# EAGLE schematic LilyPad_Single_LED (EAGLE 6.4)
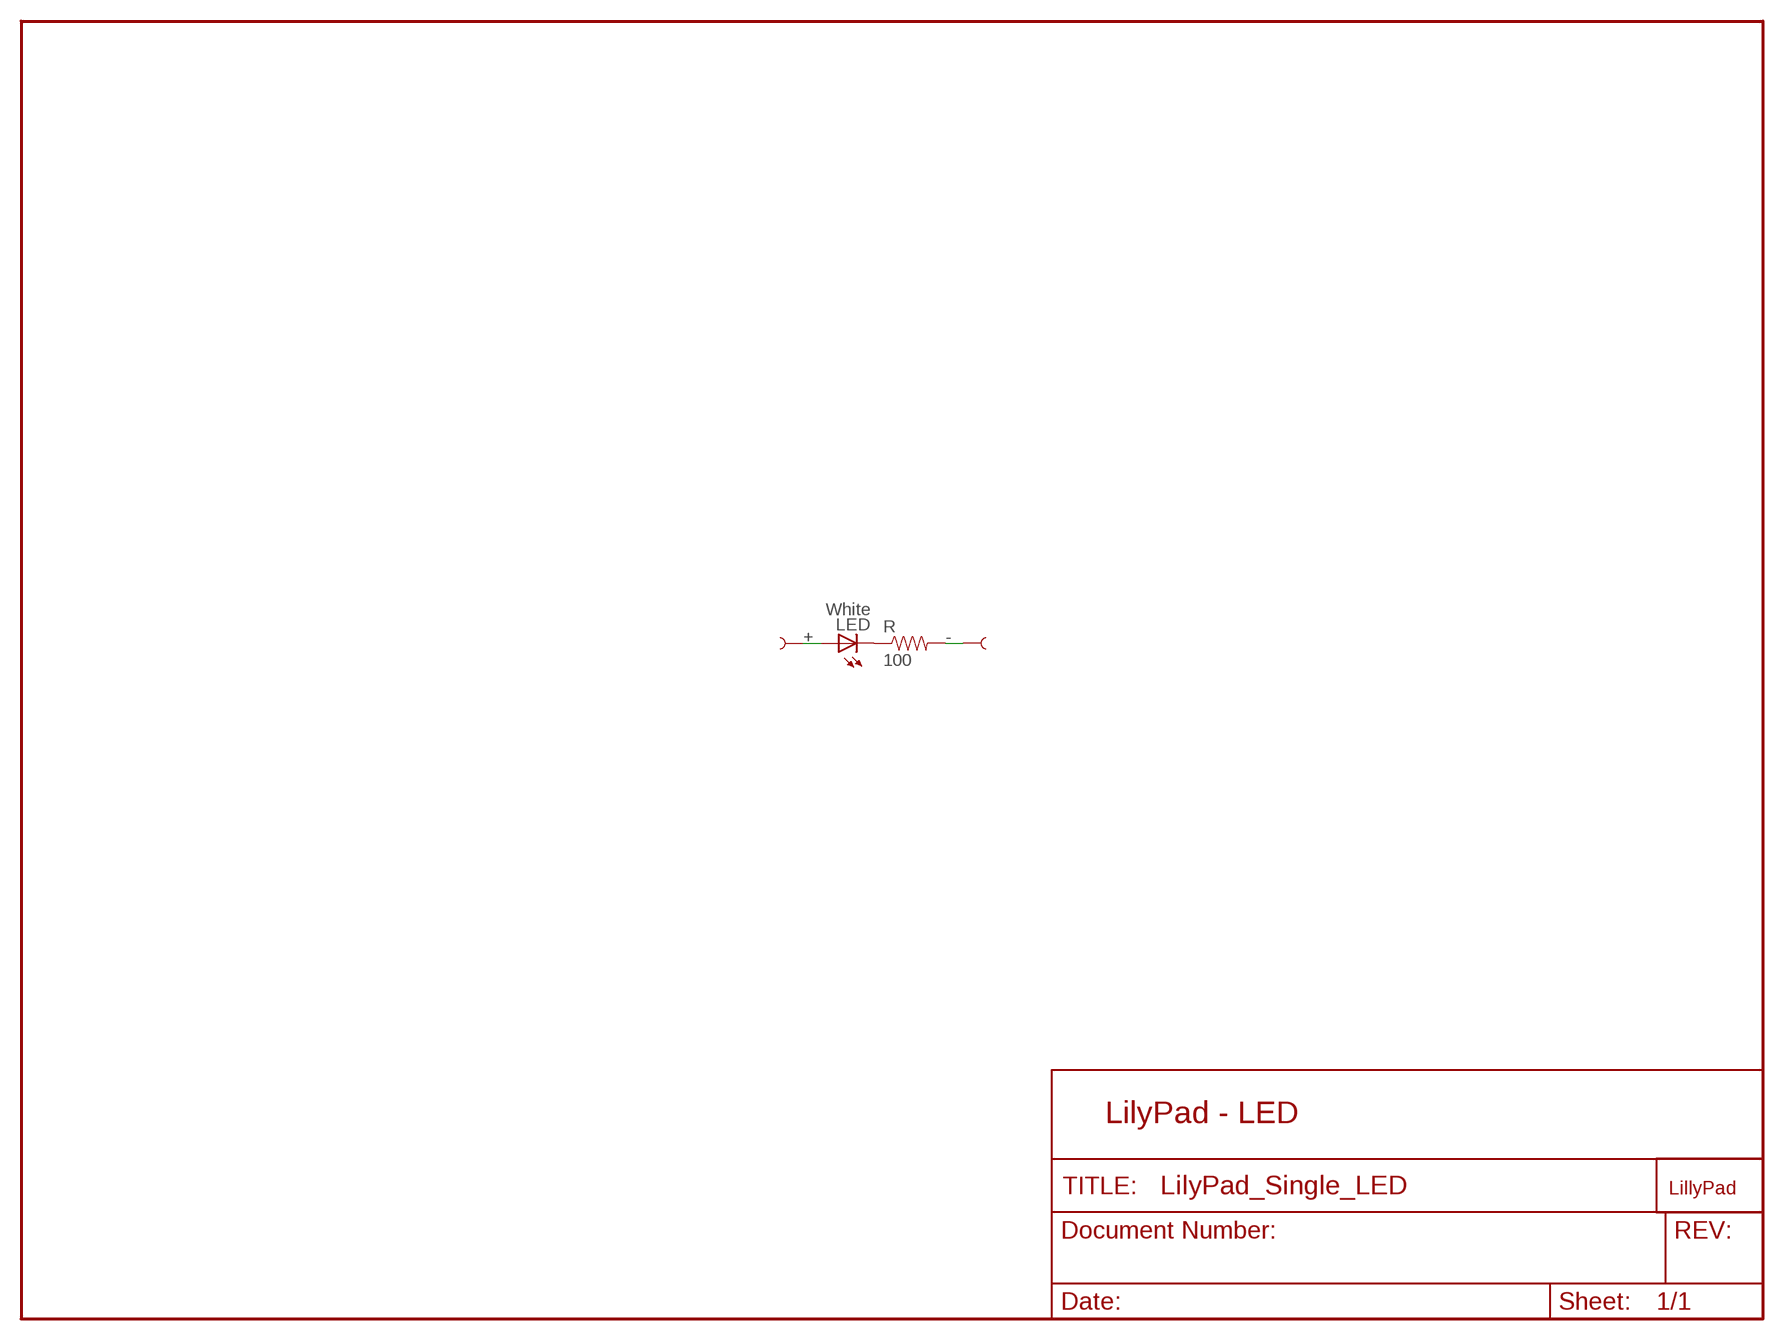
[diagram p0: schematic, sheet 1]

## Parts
LED  White  LED1206  [LED-1206]
LED+  SEWTAP6  SEWTAP4  [PETAL-SMALL]
LED-  SEWTAP6  SEWTAP2SIDE  [PETAL-SMALL]
LOGO1  LOGO-LPL  [LOGO-L]
R  100  RESISTOR0603-RES  [0603-RES]

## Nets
+: LED+.1 LED.A
-: LED-.1 R.2
N$1: LED.C R.1

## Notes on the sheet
- LilyPad - LED

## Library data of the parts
LED = SparkFun-3-2-07:LED: LEDs
LED+ LED- = LilyPad-Wearables:SEWTAP
LOGO1 = LilyPad-Wearables:LOGO-LP
R = SparkFun:RESISTOR: Resistor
